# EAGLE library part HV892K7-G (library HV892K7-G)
Display Drivers & Controllers Inductorless Liquid Lens Driver Source: Datasheet
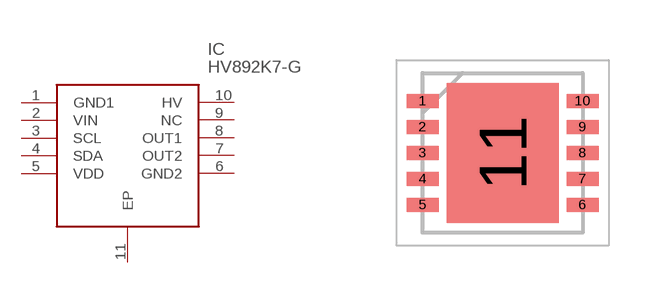
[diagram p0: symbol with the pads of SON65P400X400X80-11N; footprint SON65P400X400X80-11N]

Designator prefix IC

## HV892K7-G (Arrow_Part_Number: HV892K7-G; Arrow_Price-Stock: https://www.arrow.com/en/products/hv892k7-g/microchip-technology; Description: Display Drivers & Controllers Inductorless Liquid Lens Driver; Height: 0.8mm; Manufacturer_Name: Microchip; Manufacturer_Part_Number: HV892K7-G; Mouser_Part_Number: 689-HV892K7-G; Mouser_Price-Stock: https://www.mouser.co.uk/ProductDetail/Microchip-Technology/HV892K7-G?qs=atAAIFchRGihUhTX61zP%252BA%3D%3D)  [SON65P400X400X80-11N]
1  GND1
2  VIN
3  SCL
4  SDA
5  VDD
6  GND2
7  OUT2
8  OUT1
9  NC  nc
10  HV
11  EP

## Footprint SON65P400X400X80-11N (pad centres in mm)
10-Lead DFN Package Outline (K7)
smd 0.8 x 0.35: 1 -2,1.3; 2 -2,0.65; 3 -2,0; 4 -2,-0.65; 5 -2,-1.3; 6 2,-1.3; 7 2,-0.65; 8 2,0; 9 2,0.65; 10 2,1.3
smd 2.8 x 3.5: 11 0,0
